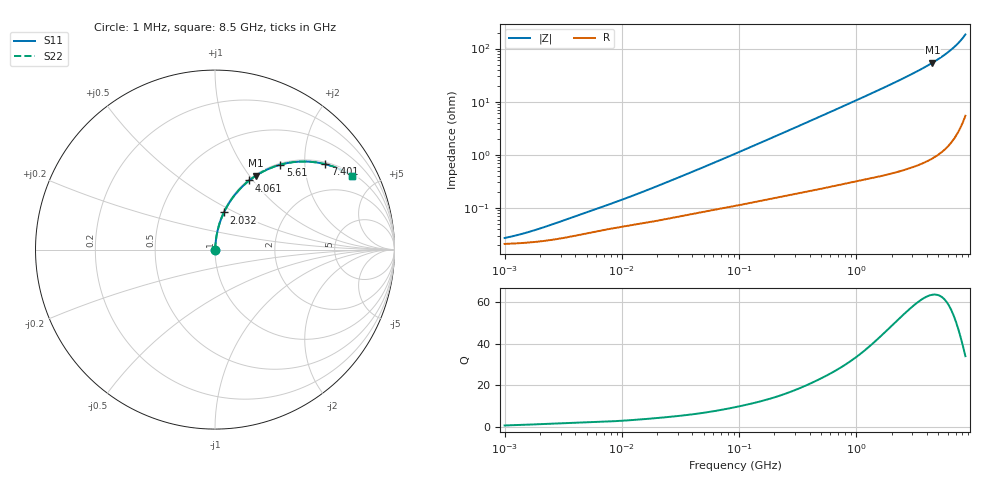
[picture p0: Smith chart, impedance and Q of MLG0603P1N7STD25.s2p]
! S-Parameter Data Generated by TDK Corporation
! Copyright(C) 2025 TDK Corporation.
! All Rights Reserved.
! TDK P/N: MLG0603P1N7STD25 (SMD / SMT Inductor (Coil))
! Property: L=1.7nH at 500MHz
! Size(LxWxT): 0.6x0.3x0.3mm
! Model Type: s2p (Touchstone File Format Version 1.0)
! Frequency: DC=Yes Start=1MHz Stop=8500MHz 198points Log-sweep
! Model Generated on Feb. 6, 2025
! Terms and conditions regarding TDK Simulation Models:
! 1)This simulation model is being provided solely for informational
!  purposes. Please refer to the specifications of the products in
!  terms of detailed characteristics of such products.
! 2)In no event shall TDK Corporation of any of its subsidiaries be
!  liable for any loss or damage arising, directly or indirectly,
!  from any information contained in this simulation model, including,
!  but not limited to loss or damages arising from any inaccuracies,
!  omissions or errors in connection with such information.
! 3)Any and all copyrights on this simulation model are owned by
!  TDK Corporation.  Duplication or redistribution of this simulation
!  model without prior written permission from TDK Corporation
!  is prohibited.
! 4)This simulation model is subject to any modification or change
!  without any prior notice.
! 5)Neither TDK Corporation nor any of its subsidiaries shall make any
!  warranty, express or implied, including but not limited to the
!  correctness, implied warranties of merchantability and fitness for
!  a particular purpose with respect to this simulation models.
! 6)The use of this simulation model shall be deemed to have consented
!  to the terms and conditions hereof.
! Port Assignments:
!  1 ---@@@--- 2
! Applicable Conditions:
!  Temperature = 25 degC
!  DC Bias Current = 0 A
!  Small Signal Operation
# Hz S MA R 50
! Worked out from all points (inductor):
!   197 points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, 1 MHz to 8.5 GHz, reference 50 ohm
!   read as one part in series: L = 2.1 nH near 9.602 MHz
!   highest Q = 63.4 at 4.454 GHz (marker M1), where L = 1.93 nH
!   S11 on the Smith chart (normalised r, x): 1 MHz: 1.00, +0.00; 2.032 GHz: 1.01, +0.44; 4.061 GHz: 1.02, +0.96; 5.61 GHz: 1.02, +1.51; 7.401 GHz: 1.05, +2.54; 8.5 GHz: 1.11, +3.68
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1000000  0.0002703 39.4  0.9998 -0.0  0.9998 -0.0  0.0002703 39.4
1319132  0.0003112 46.2  0.9998 -0.0  0.9998 -0.0  0.0003112 46.2
1822320  0.0003818 53.3  0.9998 -0.0  0.9998 -0.0  0.0003818 53.3
4587603  0.000769 65.6  0.9997 -0.0  0.9997 -0.0  0.000769 65.6
1.053054e7  0.00148 72.3  0.9996 -0.1  0.9996 -0.1  0.00148 72.3
2.10461e7  0.00268 77.3  0.9994 -0.1  0.9994 -0.1  0.00268 77.3
9.219544e7  0.01041 83.4  0.9989 -0.6  0.9989 -0.6  0.01041 83.4
4.229561e8  0.04522 84.7  0.9969 -2.6  0.9969 -2.6  0.04522 84.7
9.708683e8  0.1023 82.4  0.9917 -5.9  0.9917 -5.9  0.1023 82.4
1.404574e9  0.1474 80.1  0.9854 -8.5  0.9854 -8.5  0.1474 80.1
1.940355e9  0.2035 77.1  0.9748 -11.7  0.9748 -11.7  0.2035 77.1
2.032026e9  0.2131 76.5  0.9727 -12.3  0.9727 -12.3  0.2131 76.5
2.939772e9  0.3092 71.0  0.9456 -18.0  0.9456 -18.0  0.3092 71.0
3.535948e9  0.3731 67.2  0.9217 -21.9  0.9217 -21.9  0.3731 67.2
4.061159e9  0.4298 63.6  0.8961 -25.5  0.8961 -25.5  0.4298 63.6
4.453958e9  0.4724 60.9  0.8739 -28.2  0.8739 -28.2  0.4724 60.9
5.115526e9  0.5442 56.1  0.8304 -33.0  0.8304 -33.0  0.5442 56.1
5.610304e9  0.5974 52.4  0.7923 -36.7  0.7923 -36.7  0.5974 52.4
6.44363e9  0.6846 45.8  0.7168 -43.2  0.7168 -43.2  0.6846 45.8
7.400733e9  0.7775 37.8  0.6125 -51.0  0.6125 -51.0  0.7775 37.8
8.116539e9  0.839 31.5  0.5229 -57.0  0.5229 -57.0  0.839 31.5
8.5e9  0.8681 28.1  0.4715 -60.2  0.4715 -60.2  0.8681 28.1
